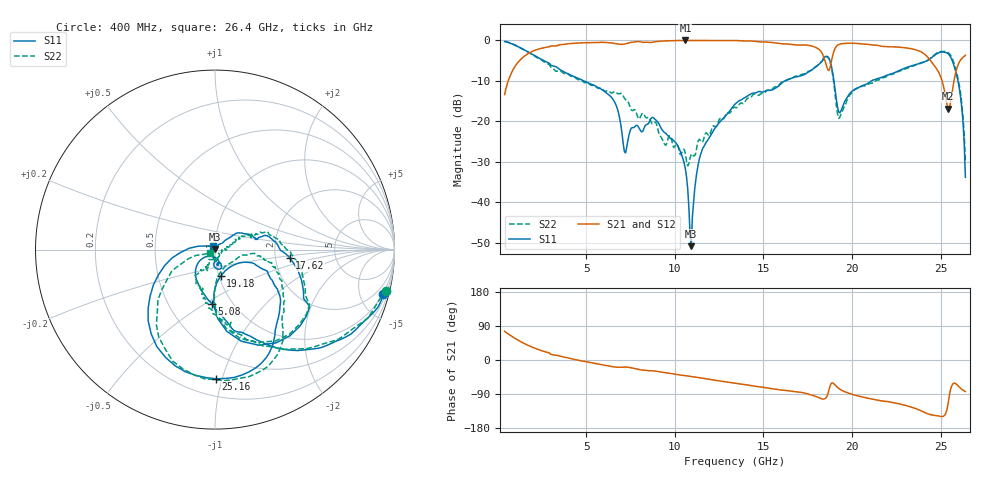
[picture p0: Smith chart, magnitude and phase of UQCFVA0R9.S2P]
!  Part Number  UQCFVA0R9  Mounting Orientation: Horizontal
!  Description: Ultra Low ESR Microwave capacitors
!  Application: Coupling, Bypass, Tuning, DC Block
!  Filters, Matching
# GHZ S DB R 50
! Freq  |S11|  S11 Ph  |S21|  S21 Ph  |S12|  S12 Ph  |S22|  S22 Ph
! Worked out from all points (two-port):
!   401 points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, 400 MHz to 26.4 GHz, reference 50 ohm
!   highest |S21| = 0.00 dB at 10.61 GHz (marker M1); lowest = -16.9 dB at 25.43 GHz (marker M2)
!   |S21| within 3 dB of the highest: 1.83 GHz to 18.29 GHz (16.46 GHz wide, 164 % of centre); 18.96 GHz to 23.97 GHz (5.016 GHz wide, 23.4 % of centre)
!   lowest |S11| = -50.8 dB at 10.93 GHz (marker M3), VSWR 1.01, Z = 49.9 + j0.28 ohm
!   |S11| at or under -10 dB: 4.872 GHz to 16.21 GHz (11.34 GHz wide, 108 % of centre); 18.98 GHz to 21.09 GHz (2.11 GHz wide, 10.5 % of centre); 25.98 GHz to end of sweep
!   |S22| runs from -31.0 to -0.2 dB; largest |S21 - S12| = 0.0077
!   S11 on the Smith chart (normalised r, x): 400 MHz: 0.93, -7.62; 5.08 GHz: 0.81, -0.53; 17.62 GHz: 2.40, -0.26; 19.18 GHz: 1.02, -0.31; 25.16 GHz: 0.32, -0.95; 26.4 GHz: 0.98, +0.03
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0.4  -0.27 -14.7  -13.36 75.6  -13.41 75.7  -0.17 -13.5
1.7  -2.77 -50.7  -3.33 39.2  -3.37 39.0  -2.82 -50.0
4.755  -9.74 -90.2  -0.60 -2.5  -0.62 -2.5  -9.88 -95.7
5.08  -10.41 -93.6  -0.55 -5.5  -0.58 -5.4  -10.41 -99.7
6.575  -14.93 -127.3  -0.70 -18.2  -0.70 -18.0  -12.68 -111.2
7.225  -27.75 -97.2  -0.83 -18.6  -0.82 -18.5  -14.61 -126.1
7.68  -21.54 -77.8  -0.40 -21.8  -0.39 -21.6  -17.15 -124.5
9.11  -20.56 -92.7  -0.21 -30.8  -0.19 -30.5  -23.04 -117.7
10.605  -31.82 -117.0  0.00 -41.5  0.00 -41.4  -28.05 -49.1
10.93  -50.79 103.6  -0.01 -43.7  -0.01 -43.6  -28.06 -29.7
11.515  -27.41 47.6  -0.01 -47.5  -0.01 -47.5  -25.14 4.5
13.4  -15.72 34.8  -0.01 -61.4  -0.01 -61.4  -16.50 27.1
17.625  -7.57 -6.2  -1.27 -91.1  -1.25 -91.3  -7.51 -2.0
17.755  -7.20 -8.7  -1.41 -92.9  -1.35 -93.0  -7.20 -5.0
18.665  -4.14 -56.8  -7.42 -85.5  -7.42 -85.5  -4.28 -56.4
19.185  -16.48 -77.7  -1.18 -72.3  -1.15 -72.6  -18.12 -74.0
22.11  -8.40 -30.3  -1.56 -110.4  -1.54 -110.7  -8.48 -20.7
24.06  -5.31 -51.0  -3.25 -137.5  -3.24 -137.8  -5.35 -46.4
25.165  -2.86 -89.6  -11.31 -148.3  -11.28 -148.6  -2.71 -82.3
25.425  -3.29 -108.8  -16.87 -114.9  -16.85 -115.4  -3.00 -99.3
26.01  -10.66 -162.6  -5.76 -69.3  -5.73 -69.6  -10.08 -148.1
26.4  -33.79 120.4  -3.69 -83.3  -3.67 -83.8  -29.81 -145.6
